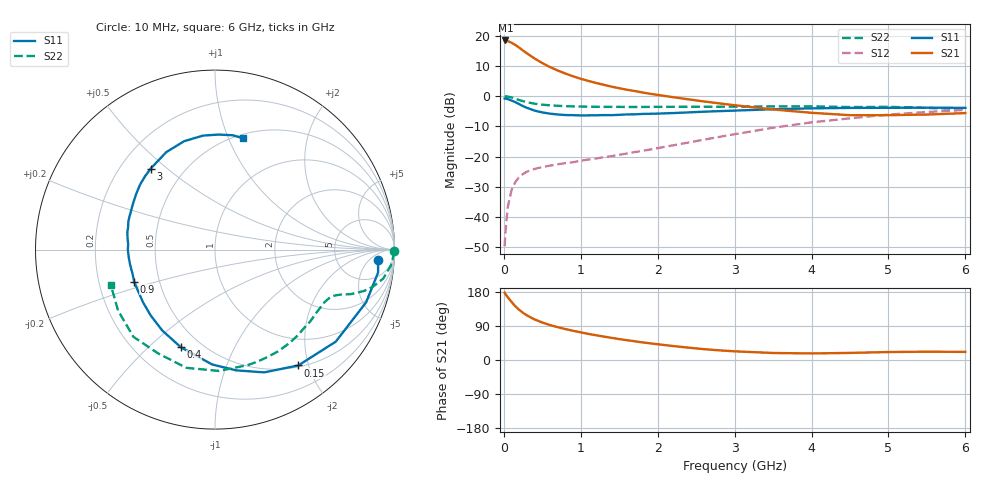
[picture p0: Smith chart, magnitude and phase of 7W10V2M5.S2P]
! Infineon Technologies  Discrete & RF Semiconductors
! BFS17W
! Si NPN RF Bipolar Junction Transistor in SOT323
! VCE = 10 V  IC = 2.5 mA
! Common Emitter S-Parameters:  August  1999
# GHz  S  MA  R  50
!  f  S11  S21  S12  S22
! GHz  MAG  ANG  MAG  ANG  MAG  ANG  MAG  ANG
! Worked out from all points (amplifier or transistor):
!   36 points, 10 MHz to 6 GHz, reference 50 ohm
!   highest |S21| = 18.4 dB at 20 MHz (marker M1)
!   |S21| within 3 dB of that: start of sweep to 232.2 MHz
!   unconditionally stable (mu >= 1): 797.6 MHz to 2.537 GHz; 5.01 GHz to end of sweep
!   at 250 MHz: K = 0.40, MSG = 20.4 dB, |S12| = -25.7 dB
!   at 1.4 GHz: K = 1.24, MAG = 8.5 dB, |S12| = -19.8 dB
!   at 6 GHz: K = 1.07, MAG = -2.1 dB, |S12| = -4.6 dB
!   S11 on the Smith chart (normalised r, x): 10 MHz: 14, -10; 150 MHz: 0.52, -1.83; 400 MHz: 0.39, -0.64; 900 MHz: 0.36, -0.17; 3 GHz: 0.33, +0.44; 6 GHz: 0.54, +1.13
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0.01  0.9105 -3.8  8.308 177.7  0.0033 84.9  0.9997 -0.6
0.02  0.9176 -8.0  8.332 174.3  0.0054 84.7  0.9941 -2.2
0.05  0.8918 -19.2  8.139 165.9  0.0144 81.0  0.9831 -5.3
0.1  0.8461 -37.3  7.644 153.4  0.0279 71.0  0.9508 -9.8
0.15  0.7949 -54.3  7.008 141.7  0.0382 62.1  0.9042 -13.2
0.2  0.7368 -68.2  6.339 132.3  0.0462 57.3  0.8619 -15.5
0.25  0.6825 -80.2  5.669 124.4  0.0516 52.6  0.8241 -17.0
0.3  0.6399 -91.5  5.103 117.7  0.0563 49.9  0.7947 -18.2
0.4  0.5764 -109.3  4.193 107.0  0.0626 46.4  0.7492 -19.5
0.5  0.5379 -123.1  3.523 98.9  0.0672 45.1  0.7225 -20.6
0.6  0.5127 -134.4  3.024 92.2  0.0709 45.6  0.7042 -21.6
0.7  0.4971 -143.7  2.654 86.6  0.0746 46.4  0.6922 -22.9
0.9  0.4845 -158.4  2.127 77.1  0.0808 49.2  0.676 -25.9
1.1  0.4804 -169.9  1.783 68.8  0.0895 52.6  0.6691 -29.3
1.3  0.4857 -179.8  1.539 61.7  0.0977 56.2  0.664 -33.3
1.6  0.4982 168.6  1.275 52.2  0.1124 61.3  0.6616 -39.5
2.2  0.5247 150.2  0.961 36.8  0.1536 69.1  0.6656 -53.6
3  0.5763 128.5  0.707 22.9  0.2345 71.7  0.6686 -73.9
3.5  0.6073 116.5  0.602 18.5  0.3001 69.2  0.6766 -88.0
4.5  0.6386 96.0  0.484 18.7  0.4296 57.7  0.6594 -118.7
5.5  0.6446 81.2  0.496 21.9  0.5463 44.0  0.638 -147.9
6  0.6399 75.7  0.524 21.4  0.5915 37.3  0.6131 -161.0
